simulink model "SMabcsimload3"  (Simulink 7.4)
settings: Solver=ode45  StartTime=0.0  StopTime=10  MaxStep=2e-4  RelTol=1e-3
InitFcn:
  | smparamload3
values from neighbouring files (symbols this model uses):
  Bm = 0.10    (= 0.1)    [IMabc2.m]    (also in imabcparam.m = 0.01; IMabcrun0.m = 0.01; IMabcrun1.m = 0.001; IMcur0.m = 1e-06)
  D = str2num(get(h,'string'))    [acttrcalc1.m]
  gam = 2*pi/3    (= 2.09439510239)    [IMabc2.m]    (also in IMabcf0.m; IMabcf1.m; imabcparam.m; IMabcrun0.m)
  H = 0.60    (= 0.6)    [IMabc2.m]    (also in IMcur0.m = 0.3; imdef0vec.m = 0.3; imdef1vec.m = 0.3; imdef2vec.m = 0.3)
  Lrr = [Lr   -Lm/2 -Lm/2    [IMabc2.m]    (also in IMabcf0.m = [Lr   -Lm1/2 -Lm1/2; IMabcf1.m = [Lr   -Lm1/2 -Lm1/2)
  Lss = [Ls   -Lm/2 -Lm/2    [IMabc2.m]    (also in IMabcf0.m = [Ls   -Lm1/2 -Lm1/2; IMabcf1.m = [Ls   -Lm1/2 -Lm1/2)
  R = str2num(get(h,'string'))    [acttrcalc1.m]    (also in IMabc2.m = diag([Rs Rs Rs Rr Rr Rr]); IMabcf0.m = diag([Rs Rs Rs Rr Rr Rr]); IMabcf1.m = diag([Rs Rs Rs Rr Rr Rr]); IMcurf0.m = diag([Rs Rs Rr Rr]))
  t1 = 2.0    (= 2)    [IMabc2.m]
  Vm = Vll*sqrt(2/3)    [imabcparam.m]
  wo = 2*pi*freq0    [calc0.m]    (also in IMabc2.m = 376.991118431; imabcparam.m = 376.991118431; IMabcrun0.m = 376.991118431; IMabcrun1.m = 376.991118431)
undefined symbols (not defined in the file or in its folder): ifo, Laf, Lakd, Lakq, Row, t2, TL1, vector, vf1, vf2

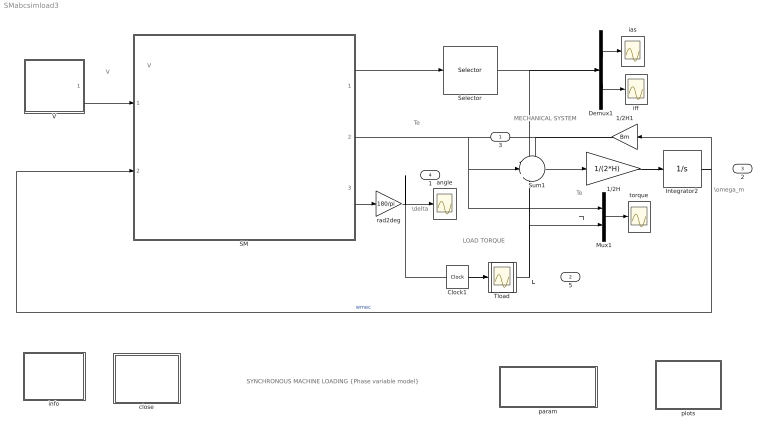
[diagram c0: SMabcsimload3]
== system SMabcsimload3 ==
  note: MECHANICAL SYSTEM
  note: SYNCHRONOUS MACHINE LOADING {Phase variable model}
  note: Te
  note: Te
  note: TL
  note: LOAD TORQUE
  note: \omega_m
  note: V
  note: I
  note: \delta
  note: TL
  note: V
  " " : Lookup  InputValues=[0 t1 9 10]  Table="[TL1 TL1  TL1-1.6 TL1-1.6]"  OutDataType=sfix(16)  OutScaling=2^0
  1/2H : Gain  Gain=1/(2*H)  ParameterDataType=sfix(16)  ParameterScaling=2^0  OutDataType=sfix(16)  OutScaling=2^0
  1/2H1 : Gain  Gain=Bm  ParameterDataType=sfix(16)  ParameterScaling=2^0  OutDataType=sfix(16)  OutScaling=2^0
  Clock1 : Clock
  Demux1 : Demux  Outputs=2
  Integrator2 : Integrator  InitialCondition=1
  Mux1 : Mux  Inputs=2
  SM : Subsystem
  Selector : Selector  InputPortWidth=6  IndexOptions=Index vector (dialog)  Indices=[1 4 ]  OutputSizes=1
  Sum1 : Sum  Inputs=-|+|-  OutDataType=sfix(16)  OutScaling=2^0
  Tload : Scope
  V : Subsystem
  angle : Scope
  close : Subsystem
  ias : Scope
  iff : Scope
  info : Subsystem
  param : Subsystem
  plots : Subsystem
  rad2deg : Gain  Gain=180/pi  ParameterDataType=sfix(16)  ParameterScaling=2^0  OutDataType=sfix(16)  OutScaling=2^0
  torque : Scope
  3 : Outport
  5 : Outport  Port=2
  2 : Outport  Port=3
  1 : Outport  Port=4
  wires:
  1/2H/1 -> Integrator2/1
  Integrator2/1 -> 1/2H1/1, SM/2(wm), 2/1  "wmec"
  V/1(V) -> SM/1(V)
  Sum1/1 -> 1/2H/1
  Mux1/1 -> torque/1
  " "/1 -> 5/1, Sum1/3, Mux1/2
  Clock1/1 -> " "/1
  Demux1/2 -> iff/1
  Demux1/1 -> ias/1
  1/2H1/1 -> Sum1/1
  SM/1(I) -> Selector/1
  Selector/1 -> Demux1/1
  SM/2(Te) -> 3/1, Sum1/2, Mux1/1
  rad2deg/1 -> angle/1, 1/1
  SM/3(delta) -> rad2deg/1

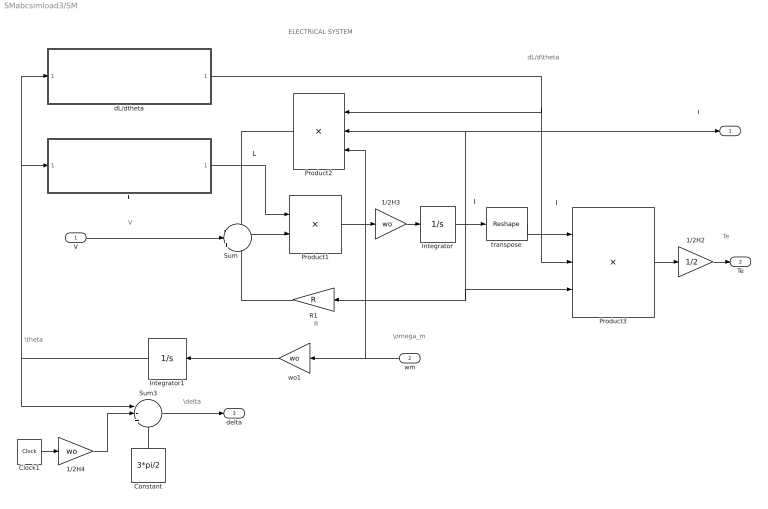
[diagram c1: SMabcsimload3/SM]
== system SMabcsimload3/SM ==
  note: \theta
  note: dL/d\theta
  note: L
  note: V
  note: ELECTRICAL SYSTEM
  note: I'
  note: I
  note: Te
  note: I
  note: \omega_m
  note: R
  note: \delta
  V : Inport  OutDataType=sfix(16)  OutScaling=2^0
  wm : Inport  Port=2  OutDataType=sfix(16)  OutScaling=2^0
  1/2H2 : Gain  Gain=1/2  ParameterDataType=sfix(16)  ParameterScaling=2^0  OutDataType=sfix(16)  OutScaling=2^0
  1/2H3 : Gain  Gain=wo  ParameterDataType=sfix(16)  ParameterScaling=2^0  OutDataType=sfix(16)  OutScaling=2^0
  1/2H4 : Gain  Gain=wo  ParameterDataType=sfix(16)  ParameterScaling=2^0  OutDataType=sfix(16)  OutScaling=2^0
  Clock1 : Clock
  Constant : Constant  Value=3*pi/2  OutDataType=sfix(16)  OutScaling=2^0
  Integrator : Integrator  InitialCondition="[-0.0133    0.0414   -0.0281    ifo   0.0000    0.0000  ]'"  ZeroCross=off
  Integrator1 : Integrator  InitialCondition=4.7323
  L : Subsystem
  Product1 : Product  Inputs=/*  Multiplication=Matrix(*)  OutDataType=sfix(16)  OutScaling=2^0
  Product2 : Product  Inputs=***  Multiplication=Matrix(*)  OutDataType=sfix(16)  OutScaling=2^0
  Product3 : Product  Inputs=3  Multiplication=Matrix(*)  OutDataType=sfix(16)  OutScaling=2^0
  R1 : Gain  Gain=R  Multiplication=Matrix(K*u)  ParameterDataType=sfix(16)  ParameterScaling=2^0  OutDataType=sfix(16)  OutScaling=2^0
  Sum : Sum  Inputs=-|+|-  OutDataType=sfix(16)  OutScaling=2^0
  Sum3 : Sum  Inputs=|-++  OutDataType=sfix(16)  OutScaling=2^0
  dL/dtheta : Subsystem
  transpose : Reshape  OutputDimensionality=Row vector (2-D)  OutputDimensions=[1,6]
  wo1 : Gain  Gain=wo  ParameterDataType=sfix(16)  ParameterScaling=2^0  OutDataType=sfix(16)  OutScaling=2^0
  I : Outport
  Te : Outport  Port=2
  delta : Outport  Port=3
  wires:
  wo1/1 -> Integrator1/1
  R1/1 -> Sum/3
  1/2H3/1 -> Integrator/1
  Integrator/1 -> transpose/1, Product2/2, I/1, R1/1, Product3/3
  L/1(L) -> Product1/1
  Integrator1/1 -> dL/dtheta/1(theta1), L/1(theta), Sum3/1
  Product3/1 -> 1/2H2/1
  dL/dtheta/1(dLdtheta) -> Product2/1, Product3/2
  Product2/1 -> Sum/1
  transpose/1 -> Product3/1
  Sum/1 -> Product1/2
  Product1/1 -> 1/2H3/1
  wm/1 -> Product2/3, wo1/1
  V/1 -> Sum/2
  1/2H2/1 -> Te/1
  Clock1/1 -> 1/2H4/1
  1/2H4/1 -> Sum3/2
  Constant/1 -> Sum3/3
  Sum3/1 -> delta/1

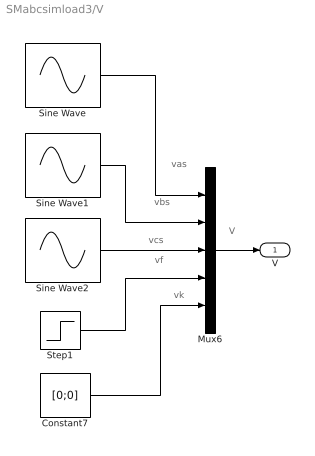
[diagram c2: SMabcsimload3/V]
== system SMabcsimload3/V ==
  note: V
  note: vf
  note: vcs
  note: vbs
  note: vas
  note: vk
  Constant7 : Constant  Value=[0;0]  VectorParams1D=off  OutDataType=sfix(16)  OutScaling=2^0
  Mux6 : Mux  Inputs=5
  Sine Wave : Sin  Amplitude=Vm  Bias=0  Frequency=wo  Phase=pi/2  Samples=10  SampleTime=0
  Sine Wave1 : Sin  Amplitude=Vm  Bias=0  Frequency=wo  Phase=pi/2-gam  Samples=10  SampleTime=0
  Sine Wave2 : Sin  Amplitude=Vm  Bias=0  Frequency=wo  Phase=pi/2+gam  Samples=10  SampleTime=0
  Step1 : Step  Time=t2  Before=vf1  After=vf2  SampleTime=0
  V : Outport
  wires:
  Mux6/1 -> V/1
  Sine Wave2/1 -> Mux6/3
  Sine Wave1/1 -> Mux6/2
  Sine Wave/1 -> Mux6/1
  Constant7/1 -> Mux6/5
  Step1/1 -> Mux6/4

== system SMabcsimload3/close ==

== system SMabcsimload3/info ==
  note: LOADING OF A SYNCHRONOUS GENERATOR Round Rotor (Phase variable model) [pu]
  note: An alternator is running at a light load when a sudden step reactive load is requested followed later by an active load command in the form of a ramp. The dynamic equations are expressed in matrix form in terms the phase variables, namely the stator currents ias, ibs, ics; the rotor field current iff; the d-axis and q-axis damper currents idk and iqk; the angular speed wm; and the displacement angle theta between stator as-axis and rotor direct axis. Torque, speed, and current responses are plotted including the torque angle and power factor. A Matlab script file for the identical system operation is given in the file >.

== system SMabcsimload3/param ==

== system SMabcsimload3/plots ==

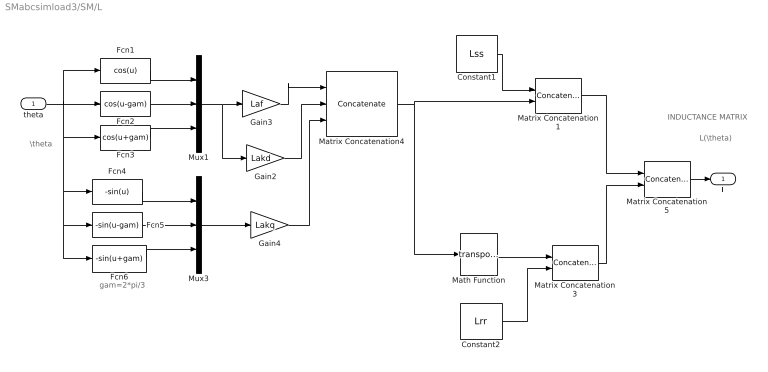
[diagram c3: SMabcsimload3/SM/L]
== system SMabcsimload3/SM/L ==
  note: INDUCTANCE MATRIX
  note: gam=2*pi/3
  note: \theta
  note: L(\theta)
  theta : Inport  OutDataType=sfix(16)  OutScaling=2^0
  Constant1 : Constant  Value=Lss  VectorParams1D=off  OutDataType=sfix(16)  OutScaling=2^0
  Constant2 : Constant  Value=Lrr  VectorParams1D=off  OutDataType=sfix(16)  OutScaling=2^0
  Fcn1 : Fcn  Expr=cos(u)
  Fcn2 : Fcn  Expr=cos(u-gam)
  Fcn3 : Fcn  Expr=cos(u+gam)
  Fcn4 : Fcn  Expr=-sin(u)
  Fcn5 : Fcn  Expr=-sin(u-gam)
  Fcn6 : Fcn  Expr=-sin(u+gam)
  Gain2 : Gain  Gain=Lakd  ParameterDataType=sfix(16)  ParameterScaling=2^0  OutDataType=sfix(16)  OutScaling=2^0
  Gain3 : Gain  Gain=Laf  ParameterDataType=sfix(16)  ParameterScaling=2^0  OutDataType=sfix(16)  OutScaling=2^0
  Gain4 : Gain  Gain=Lakq  ParameterDataType=sfix(16)  ParameterScaling=2^0  OutDataType=sfix(16)  OutScaling=2^0
  Math Function : Math  Operator=transpose
  Matrix Concatenation1 : Concatenate  Mode=Multidimensional array  ConcatenateDimension=2
  Matrix Concatenation3 : Concatenate  Mode=Multidimensional array  ConcatenateDimension=2
  Matrix Concatenation4 : Concatenate  NumInputs=3  Mode=Multidimensional array  ConcatenateDimension=2
  Matrix Concatenation5 : Concatenate  Mode=Multidimensional array
  Mux1 : Mux  Inputs=3
  Mux3 : Mux  Inputs=3
  L : Outport
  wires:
  Matrix Concatenation5/1 -> L/1
  Matrix Concatenation4/1 -> Matrix Concatenation1/2, Math Function/1
  Mux1/1 -> Gain3/1, Gain2/1
  Matrix Concatenation1/1 -> Matrix Concatenation5/1
  Constant1/1 -> Matrix Concatenation1/1
  Fcn3/1 -> Mux1/3
  Fcn2/1 -> Mux1/2
  Fcn1/1 -> Mux1/1
  theta/1 -> Fcn2/1, Fcn1/1, Fcn3/1, Fcn6/1, Fcn5/1, Fcn4/1
  Gain3/1 -> Matrix Concatenation4/1
  Gain2/1 -> Matrix Concatenation4/2
  Fcn5/1 -> Mux3/2
  Fcn4/1 -> Mux3/1
  Fcn6/1 -> Mux3/3
  Mux3/1 -> Gain4/1
  Gain4/1 -> Matrix Concatenation4/3
  Math Function/1 -> Matrix Concatenation3/1
  Constant2/1 -> Matrix Concatenation3/2
  Matrix Concatenation3/1 -> Matrix Concatenation5/2

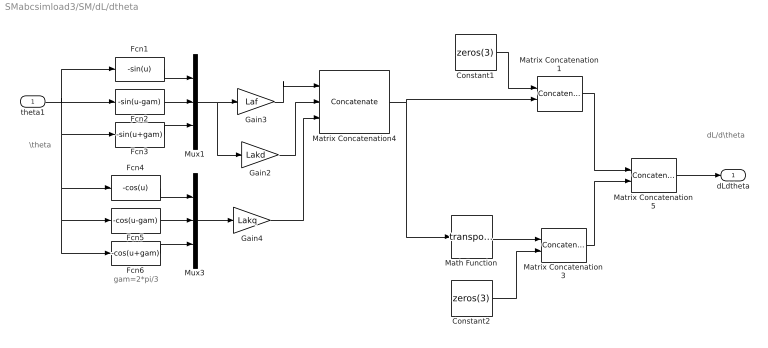
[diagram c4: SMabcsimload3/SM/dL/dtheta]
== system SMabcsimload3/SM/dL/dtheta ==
  note: dL/d\theta
  note: gam=2*pi/3
  note: \theta
  theta1 : Inport  OutDataType=sfix(16)  OutScaling=2^0
  Constant1 : Constant  Value=zeros(3)  VectorParams1D=off  OutDataType=sfix(16)  OutScaling=2^0
  Constant2 : Constant  Value=zeros(3)  VectorParams1D=off  OutDataType=sfix(16)  OutScaling=2^0
  Fcn1 : Fcn  Expr=-sin(u)
  Fcn2 : Fcn  Expr=-sin(u-gam)
  Fcn3 : Fcn  Expr=-sin(u+gam)
  Fcn4 : Fcn  Expr=-cos(u)
  Fcn5 : Fcn  Expr=-cos(u-gam)
  Fcn6 : Fcn  Expr=-cos(u+gam)
  Gain2 : Gain  Gain=Lakd  ParameterDataType=sfix(16)  ParameterScaling=2^0  OutDataType=sfix(16)  OutScaling=2^0
  Gain3 : Gain  Gain=Laf  ParameterDataType=sfix(16)  ParameterScaling=2^0  OutDataType=sfix(16)  OutScaling=2^0
  Gain4 : Gain  Gain=Lakq  ParameterDataType=sfix(16)  ParameterScaling=2^0  OutDataType=sfix(16)  OutScaling=2^0
  Math Function : Math  Operator=transpose
  Matrix Concatenation1 : Concatenate  Mode=Multidimensional array  ConcatenateDimension=2
  Matrix Concatenation3 : Concatenate  Mode=Multidimensional array  ConcatenateDimension=2
  Matrix Concatenation4 : Concatenate  NumInputs=3  Mode=Multidimensional array  ConcatenateDimension=2
  Matrix Concatenation5 : Concatenate  Mode=Multidimensional array
  Mux1 : Mux  Inputs=3
  Mux3 : Mux  Inputs=3
  dLdtheta : Outport
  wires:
  Matrix Concatenation5/1 -> dLdtheta/1
  Matrix Concatenation4/1 -> Matrix Concatenation1/2, Math Function/1
  Mux1/1 -> Gain3/1, Gain2/1
  Matrix Concatenation1/1 -> Matrix Concatenation5/1
  Constant1/1 -> Matrix Concatenation1/1
  Fcn3/1 -> Mux1/3
  Fcn2/1 -> Mux1/2
  Fcn1/1 -> Mux1/1
  theta1/1 -> Fcn2/1, Fcn1/1, Fcn3/1, Fcn6/1, Fcn5/1, Fcn4/1
  Gain3/1 -> Matrix Concatenation4/1
  Gain2/1 -> Matrix Concatenation4/2
  Fcn5/1 -> Mux3/2
  Fcn4/1 -> Mux3/1
  Fcn6/1 -> Mux3/3
  Mux3/1 -> Gain4/1
  Gain4/1 -> Matrix Concatenation4/3
  Math Function/1 -> Matrix Concatenation3/1
  Constant2/1 -> Matrix Concatenation3/2
  Matrix Concatenation3/1 -> Matrix Concatenation5/2
